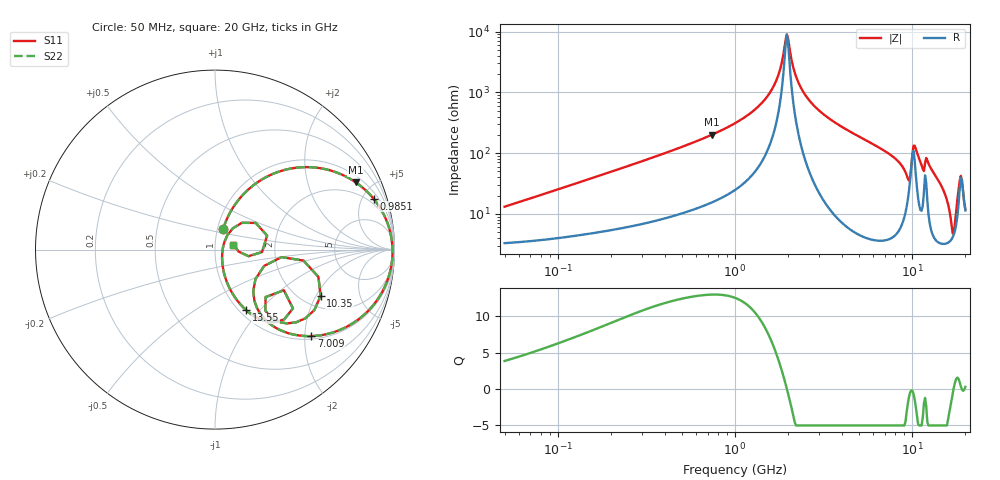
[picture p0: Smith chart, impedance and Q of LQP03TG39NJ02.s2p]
!Murata Part Number: LQP03TG39NJ02
!These Parameters are Measured in Series Mode Connection
!  o--[Z]--o
!Port1  Port2
!  o-------o
!Freq. Start=50[MHz] Stop=20[GHz], 401[Steps]
# Hz S RI R 50
!Freq.(Hz) S11(Real) S11(Imag) S21(Real) S21(Imag) S12(Real) S12(Imag) S22(Real) S22(Imag)
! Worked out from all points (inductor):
!   401 points, 50 MHz to 20 GHz, reference 50 ohm
!   read as one part in series: L = 40.1 nH near 51.52 MHz
!   highest Q = 13 at 741.1 MHz (marker M1), where L = 43 nH
!   self-resonance near 1.962 GHz
!   S11 on the Smith chart (normalised r, x): 50 MHz: 1.07, +0.25; 985.1 MHz: 1.48, +6.03; 7.009 GHz: 1.07, -2.16; 10.35 GHz: 2.49, -2.18; 13.55 GHz: 1.07, -0.85; 20 GHz: 1.23, +0.07
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5e7  0.0462 0.1171  0.9538 -0.1171  0.9538 -0.1171  0.0462 0.1171
1.364002e8  0.1333 0.2797  0.8667 -0.2797  0.8667 -0.2797  0.1333 0.2797
3.721004e8  0.4616 0.4572  0.5384 -0.4572  0.5384 -0.4572  0.4616 0.4572
7.411344e8  0.7836 0.375  0.2164 -0.375  0.2164 -0.375  0.7836 0.375
9.85133e8  0.8833 0.2838  0.1167 -0.2838  0.1167 -0.2838  0.8833 0.2838
1e9  0.8876 0.2784  0.1124 -0.2784  0.1124 -0.2784  0.8876 0.2784
1.590961e9  0.9775 0.092  0.0225 -0.092  0.0225 -0.092  0.9775 0.092
1.766834e9  0.9855 0.0466  0.0145 -0.0466  0.0145 -0.0466  0.9855 0.0466
1.962148e9  0.989 0.0005  0.011 -0.0005  0.011 -0.0005  0.989 0.0005
2.245319e9  0.9866 -0.0596  0.0134 0.0596  0.0134 0.0596  0.9866 -0.0596
2.728004e9  0.9686 -0.1477  0.0314 0.1477  0.0314 0.1477  0.9686 -0.1477
7.009217e9  0.5375 -0.482  0.4625 0.482  0.4625 0.482  0.5375 -0.482
7.442007e9  0.4821 -0.4802  0.5179 0.4802  0.5179 0.4802  0.4821 -0.4802
9.316812e9  0.2193 -0.2849  0.7807 0.2849  0.7807 0.2849  0.2193 -0.2849
9.892087e9  0.3706 -0.0418  0.6294 0.0418  0.6294 0.0418  0.3706 -0.0418
1.034674e10  0.5883 -0.2576  0.4117 0.2576  0.4117 0.2576  0.5883 -0.2576
1.098561e10  0.4018 -0.4111  0.5982 0.4111  0.5982 0.4111  0.4018 -0.4111
1.354865e10  0.1735 -0.3371  0.8265 0.3371  0.8265 0.3371  0.1735 -0.3371
1.550395e10  0.063 -0.1723  0.937 0.1723  0.937 0.1723  0.063 -0.1723
1.696185e10  0.0401 -0.0214  0.9599 0.0214  0.9599 0.0214  0.0401 -0.0214
1.855685e10  0.2269 0.1487  0.7731 -0.1487  0.7731 -0.1487  0.2269 0.1487
2e10  0.1028 0.0277  0.8972 -0.0277  0.8972 -0.0277  0.1028 0.0277
